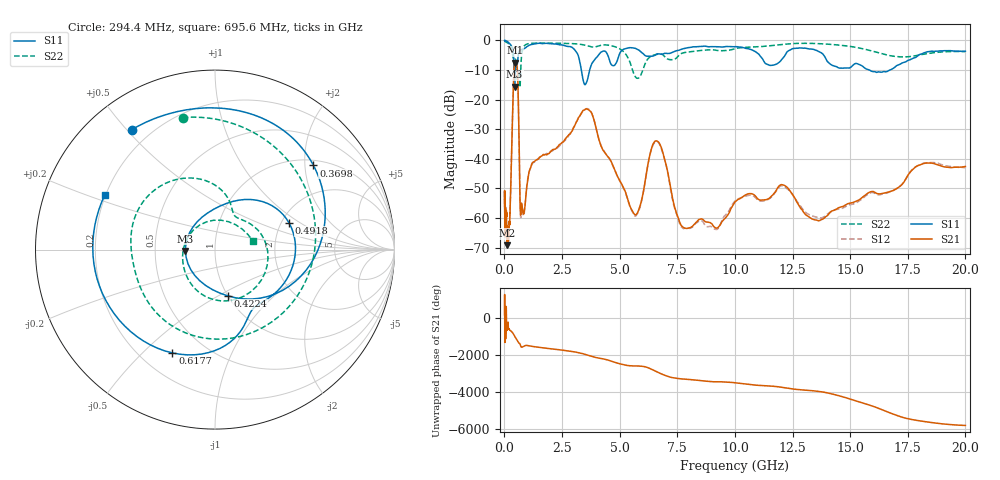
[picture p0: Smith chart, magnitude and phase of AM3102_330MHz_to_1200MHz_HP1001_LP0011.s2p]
! Date/Time: Tue, Sep 11, 2018 5:17 PM
! Network Analyzer: Agilent Technologies E8362B Rev: A.07.50.63
! Sweep from 0.010 to 20.000 GHz, 1601 Points, Sweep Type: LOG
! Power Supply: 4.949 V, 0.001 A
# Hz S DB R 50
!freq MagS11 AngS11 MagS21 AngS21 MagS12 AngS12 MagS22 AngS22
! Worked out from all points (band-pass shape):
!   1601 points, 10 MHz to 20 GHz, reference 50 ohm
!   highest |S21| = -7.50 dB at 462.3 MHz (marker M1); lowest = -69.2 dB at 111.2 MHz (marker M2)
!   |S21| within 3 dB of the highest: 414.6 MHz to 567.2 MHz (152.6 MHz wide, 31.1 % of centre)
!   lowest |S11| = -15.7 dB at 440.9 MHz (marker M3), VSWR 1.39, Z = 35.9 - j0.56 ohm
!   |S11| at or under -10 dB: 418.6 MHz to 467.9 MHz (49.3 MHz wide, 11.1 % of centre); 3.34 GHz to 3.7 GHz (360.3 MHz wide, 10.2 % of centre); 15.84 GHz to 16.72 GHz (882.3 MHz wide, 5.42 % of centre)
!   |S22| runs from -15.8 to -0.1 dB; largest |S21 - S12| = 0.0051
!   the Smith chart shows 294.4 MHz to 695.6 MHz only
!   S11 on the Smith chart (normalised r, x): 294.4 MHz: 0.13, +0.52; 369.8 MHz: 1.13, +2.21; 422.4 MHz: 1.00, -0.55; 491.8 MHz: 2.20, +0.81; 617.7 MHz: 0.33, -0.62; 695.6 MHz: 0.20, +0.22
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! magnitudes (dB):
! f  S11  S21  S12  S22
! 10 MHz  0.0  -51.0  -56.8  -0.1
! 35.55 MHz  0.0  -62.7  -64.0  -0.3
! 83.6 MHz  -0.2  -57.7  -65.6  -0.6
! 111.2 MHz  -0.3  -69.2  -63.9  -0.7
! 126.4 MHz  -0.4  -67.4  -64.4  -0.8
! 203.3 MHz  -1.0  -63.1  -64.3  -1.2
! 294.4 MHz  -1.8  -43.9  -44.0  -2.4
! 369.8 MHz  -2.8  -20.8  -20.9  -5.5
! 422.4 MHz  -11.5  -9.4  -9.5  -6.5
! 440.9 MHz  -15.7  -7.9  -7.9  -6.7
! 447.2 MHz  -15.4  -7.7  -7.7  -6.7
! 462.3 MHz  -11.5  -7.5  -7.6  -6.5
! 491.8 MHz  -7.2  -7.7  -7.7  -6.5
! 617.7 MHz  -4.1  -25.3  -25.3  -10.2
! 695.6 MHz  -3.3  -58.2  -59.0  -13.2
! 1.59 GHz  -1.0  -39.1  -39.1  -0.9
! 3.634 GHz  -12.3  -23.3  -23.1  -1.9
! 5.652 GHz  -2.6  -58.8  -59.3  -11.9
! 6.58 GHz  -4.7  -33.9  -34.1  -4.8
! 7.92 GHz  -2.5  -63.5  -63.5  -4.0
! 13.68 GHz  -3.9  -60.9  -59.9  -1.1
! 20 GHz  -3.6  -42.6  -43.0  -3.7
